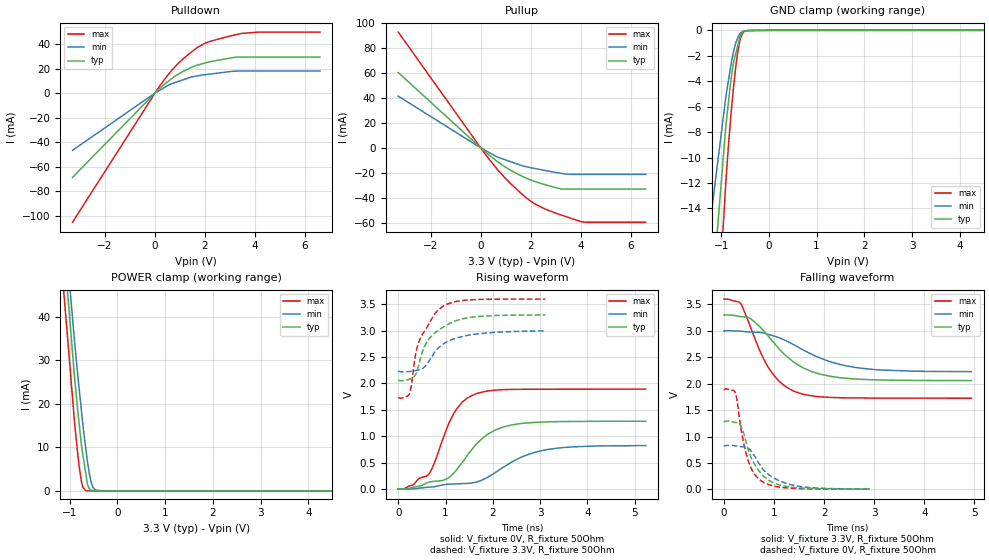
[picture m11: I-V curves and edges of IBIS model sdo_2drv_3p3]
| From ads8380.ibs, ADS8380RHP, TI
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|   sdo_2drv_3p3 Model
[Model]   sdo_2drv_3p3
Model_type   3-state
Polarity   Non-Inverting
Vmeas = 1.65
Vref = 1.65
Cref = 10pF
Rref = 50
|   typ   min   max
|   (nom PVT)   (fast PVT)   (slow PVT)
|C_comp from frequency sweep method (F=40MHz)
C_comp   5.373e-12   5.292e-12   5.471e-12
|ON state : BUFFER OUTPUT TURNED HIGH
|C_comp   5.373e-12   5.292e-12   5.471e-12
|OFF state: BUFFER IN HIGH IMPEDANCE
|C_comp   5.648e-12   5.537e-12   5.708e-12
|C_comp from LC tank measurement(L=1nH)
|Resonant Frequency(Hz)   3.960e+09   3.970e+09   3.900e+09
|C_comp   1.617e-12   1.609e-12   1.667e-12
|ON state : BUFFER OUTPUT TURNED HIGH
|Resonant Frequency(Hz)   3.960e+09   3.970e+09   3.900e+09
|C_comp   1.617e-12   1.609e-12   1.667e-12
|OFF state: BUFFER IN HIGH IMPEDANCE
|Resonant Frequency(Hz)   3.970e+09   3.990e+09   3.910e+09
|C_comp   1.609e-12   1.593e-12   1.659e-12
| Where nom  PVT is Nominal Process, 3.3V, 35C
|   Fast PVT is Strong Process,  3.6V, -40C
|   Slow PVT is Weak Process,   3V, 95C
[Voltage Range]   3.3   3   3.6
|Ambient Temperature   25   85   -40
|Junction Temperature
[Temperature Range]   35   95   -40
[Pullup Reference]   3.3   3   3.6
[Pulldown Reference]   0   0   0
[Power Clamp Reference]   3.3   3   3.6
[GND Clamp Reference]   0   0   0
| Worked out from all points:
|   slope of the pulldown table from 0 to 0.495 V, typ, clamps not added: 54.8 ohm
|   slope of the pullup table from 0 to 0.495 V, typ, clamps not added: 59.7 ohm
|   GND clamp passes 1 mA (typ) near -0.64 V on its own axis
|   POWER clamp passes 1 mA (typ) near -0.61 V on its own axis
|   falling waveform, V_fixture 3.3V, R_fixture 50Ohm: 20-80 % time 825ps typ, 1.08ns min, 582ps max; typ from 3.3 V to 2.06 V
|   rising waveform, V_fixture 0V, R_fixture 50Ohm: 20-80 % time 753ps typ, 1ns min, 527ps max; typ from 0 V to 1.28 V
|   rising waveform, V_fixture 3.3V, R_fixture 50Ohm: 20-80 % time 503ps typ, 551ps min, 410ps max; typ from 2.05 V to 3.3 V
|   falling waveform, V_fixture 0V, R_fixture 50Ohm: 20-80 % time 377ps typ, 500ps min, 267ps max; typ from 1.29 V to 0.004 V
[Pulldown]
|   Voltage   I(typ)   I(min)   I(max)
-3.3V     -68.58mA   -46.56mA   -105.1mA
208.8mV   4.11mA     2.527mA    6.379mA
633mV     11.3mA     7.445mA    17.64mA
939.6mV   15.49mA    9.557mA    24.39mA
1.464V    20.97mA    13.17mA    33.49mA
1.706V    22.82mA    14.05mA    37.32mA
2.203V    25.53mA    15.48mA    42.06mA
3.267V    29.34mA    17.92mA    47.69mA
3.449V    29.34mA    17.98mA    48.53mA
4.162V    29.34mA    17.99mA    49.65mA
6.6V      29.34mA    17.99mA    49.65mA
[GND Clamp]
|   Voltage   I(typ)   I(min)   I(max)
-3.3V     -300mA     -183.9mA   -660.5mA
-1.573V   -38.55mA   -27.45mA   -59mA
-1.224V   -22.44mA   -14.97mA   -32.48mA
-897.6mV  -7.374mA   -5.135mA   -11.71mA
-842.4mV  -5.499mA   -3.836mA   -8.853mA
-792mV    -3.869mA   -2.653mA   -6.546mA
-745.8mV  -2.607mA   -1.779mA   -4.695mA
-687.6mV  -1.73mA    -926.9uA   -2.685mA
-640.8mV  -1.025mA   -506uA     -1.451mA
-601.2mV  -429uA     -239.4uA   -723uA
-519mV    -57.29uA   -42.94uA   -108.9uA
6.6V      0A         0A         0A
[Pullup]
|   Voltage   I(typ)   I(min)   I(max)
-3.3V     60.17mA    41.29mA    92.47mA
18mV      -318.2uA   -221.2uA   -502.9uA
478.8mV   -8.039mA   -5.335mA   -12.67mA
702mV     -11.45mA   -7.642mA   -18.04mA
1.228V    -18.24mA   -11.29mA   -29.18mA
1.861V    -24.56mA   -15.28mA   -40.5mA
2.167V    -26.92mA   -16.51mA   -44.76mA
2.473V    -28.83mA   -17.69mA   -47.94mA
3.241V    -32.95mA   -20.45mA   -53.77mA
4.032V    -32.95mA   -21.18mA   -58.99mA
6.6V      -32.95mA   -21.18mA   -59.39mA
[POWER Clamp]
|   Voltage   I(typ)   I(min)   I(max)
-3.3V     597.5mA    489.1mA    865.1mA
-1.156V   60.55mA    67.18mA    49.96mA
-897.6mV  26.03mA    34.25mA    15.65mA
-824.4mV  17.75mA    25.92mA    7.74mA
-766.8mV  11.86mA    19.74mA    2.964mA
-720mV    7.952mA    14.91mA    731.1uA
-662.4mV  3.944mA    9.643mA    56.93uA
-627mV    1.481mA    6.651mA    11.79uA
-549mV    129uA      1.968mA    6.895uA
-510mV    73.36uA    791.2uA    4.446uA
-462mV    4.874uA    205uA      1.433uA
6.6V      0A         0A         0A
[Ramp]
R_load = 50
|   typ   min   max
dV/dt_r   0.773357/7.56731e-10   0.496661/1.00831e-09   1.1373/5.26054e-10
dV/dt_f   0.74753/8.29607e-10   0.466045/1.08848e-09   1.12625/5.83316e-10
[Falling Waveform]
V_fixture = 3.3V
V_fixture_min = 3V
V_fixture_max = 3.6V
R_fixture = 50Ohm
|   Time   V(typ)   V(min)   V(max)
0s        3.3V       3V         3.6V
342ps     3.268V     2.992V     3.504V
538ps     3.225V     2.976V     3.051V
742ps     3.052V     2.966V     2.568V
898ps     2.884V     2.928V     2.29V
1.132ns   2.629V     2.857V     2.022V
1.406ns   2.398V     2.73V      1.854V
1.92ns    2.18V      2.484V     1.752V
2.566ns   2.091V     2.316V     1.73V
4.94ns    2.058V     2.227V     1.725V
[Rising Waveform]
V_fixture = 0V
V_fixture_min = 0V
V_fixture_max = 0V
R_fixture = 50Ohm
|   Time   V(typ)   V(min)   V(max)
0s        3.488nV    7.586nV    3.033nV
642ps     129.8mV    36mV       278.4mV
760ps     147.3mV    44.99mV    482mV
942ps     165.3mV    80.22mV    944.7mV
1.16ns    289.3mV    97.3mV     1.406V
1.354ns   503.6mV    103.4mV    1.647V
1.642ns   841.2mV    130.7mV    1.804V
2.216ns   1.173V     409.4mV    1.882V
3.14ns    1.272V     746.8mV    1.89V
5.234ns   1.285V     824mV      1.893V
[Rising Waveform]
V_fixture = 3.3V
V_fixture_min = 3V
V_fixture_max = 3.6V
R_fixture = 50Ohm
|   Time   V(typ)   V(min)   V(max)
0s        2.054V     2.223V     1.723V
234ps     2.08V      2.226V     1.797V
276ps     2.093V     2.23V      1.951V
368ps     2.171V     2.245V     2.547V
450ps     2.401V     2.261V     2.818V
616ps     2.802V     2.374V     3.075V
786ps     2.964V     2.61V      3.333V
972ps     3.076V     2.759V     3.474V
1.674ns   3.265V     2.937V     3.589V
3.112ns   3.296V     2.994V     3.597V
[Falling Waveform]
V_fixture = 0V
V_fixture_min = 0V
V_fixture_max = 0V
R_fixture = 50Ohm
|   Time   V(typ)   V(min)   V(max)
0s        1.289V     828.3mV    1.896V
226ps     1.267V     824.3mV    1.838V
268ps     1.261V     818.6mV    1.639V
350ps     1.178V     808mV      1.088V
478ps     769mV      777.9mV    566.4mV
586ps     520.1mV    668.6mV    324.2mV
734ps     308.6mV    439.7mV    167.4mV
1.05ns    102mV      187.5mV    52.05mV
1.416ns   34.51mV    70.21mV    17.81mV
2.916ns   4.421mV    4.573mV    3.878mV
